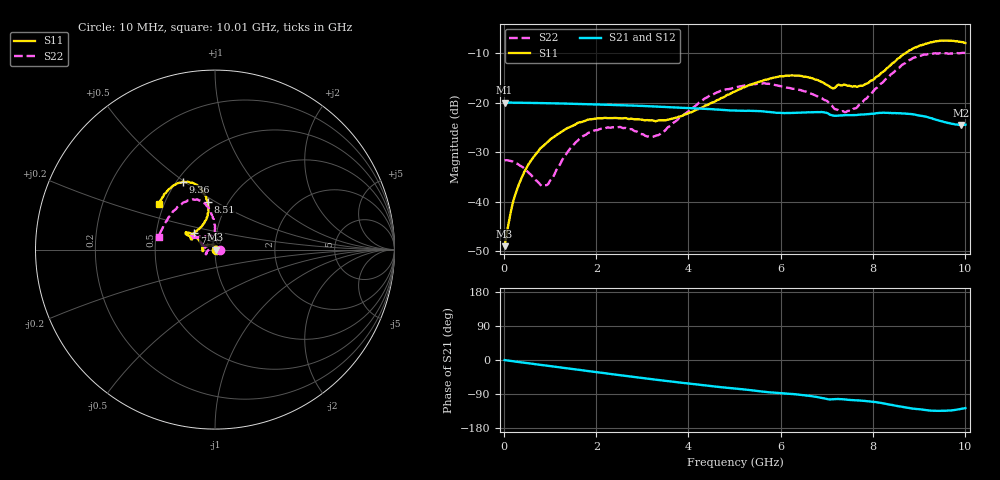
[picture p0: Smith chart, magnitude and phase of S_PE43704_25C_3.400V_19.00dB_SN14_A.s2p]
! Device ID: PE43704
! Dir: z:\PE43704\PE43704_Char_1_20130516\PE43704\AMB\3p400V\19p00dB
! Serial: 14
! Insertion: A
! Impedance: 50 ohm
! Temp: Amb
! VDD: 3.400V
! Attenuation Step: 19.00dB
! IDD: 1.140463e-01mA
#  Hz  S  RI  R  50
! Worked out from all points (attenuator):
!   401 points, 10 MHz to 10.01 GHz, reference 50 ohm
!   highest |S21| = -19.96 dB at 10 MHz (marker M1); lowest = -24.5 dB at 9.91 GHz (marker M2)
!   lowest |S11| = -49.0 dB at 10 MHz (marker M3), VSWR 1.01, Z = 50.4 + j0.047 ohm
!   |S11| at or under -10 dB: start of sweep to 8.714 GHz
!   |S22| runs from -36.9 to -9.9 dB; largest |S21 - S12| = 0.0012
!   S11 on the Smith chart (normalised r, x): 10 MHz: 1.01, +0.00; 7.46 GHz: 0.78, +0.15; 8.51 GHz: 0.81, +0.46; 9.36 GHz: 0.54, +0.49; 10.01 GHz: 0.47, +0.28
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1e7  0.00352 0.000467  0.1005 -0.000334  0.1005 -0.000251  0.0261 0.000237
2.35e8  0.00173 0.0114  0.0999 -0.00701  0.0999 -0.00697  0.0237 0.0071
5.6e8  -0.00776 0.0238  0.0983 -0.0161  0.0982 -0.0161  0.0133 0.0138
8.1e8  -0.0198 0.0293  0.0964 -0.0229  0.0964 -0.0229  0.000923 0.0145
9.35e8  -0.0261 0.0297  0.0953 -0.0262  0.0953 -0.0261  -0.00619 0.0134
1.385e9  -0.0504 0.024  0.0903 -0.0375  0.0904 -0.0375  -0.0321 0.00166
1.685e9  -0.062 0.0152  0.0862 -0.0445  0.0863 -0.0445  -0.0441 -0.00997
2.385e9  -0.0699 -0.00424  0.0747 -0.0585  0.0747 -0.0585  -0.0507 -0.0253
3.36e9  -0.0664 -0.000702  0.0549 -0.0728  0.055 -0.0727  -0.0473 0.00192
4.385e9  -0.084 0.0429  0.0334 -0.0801  0.0334 -0.0802  -0.0947 0.0598
5.01e9  -0.1083 0.0719  0.0212 -0.0807  0.0213 -0.0806  -0.1224 0.0733
5.96e9  -0.1565 0.0955  0.00392 -0.079  0.0042 -0.0789  -0.128 0.0741
6.685e9  -0.1565 0.0818  -0.00812 -0.0797  -0.00818 -0.0797  -0.1011 0.0688
7.11e9  -0.1258 0.0647  -0.0178 -0.0726  -0.0179 -0.0726  -0.0565 0.0747
7.46e9  -0.1148 0.094  -0.0194 -0.0724  -0.0191 -0.0725  -0.0217 0.0798
7.835e9  -0.0684 0.1379  -0.024 -0.0726  -0.024 -0.0725  -0.0016 0.1084
8.36e9  -0.0366 0.2304  -0.0363 -0.0697  -0.0363 -0.0704  -0.0129 0.185
8.51e9  -0.0394 0.2657  -0.0401 -0.0672  -0.04 -0.0677  -0.025 0.2137
8.935e9  -0.0897 0.3513  -0.0479 -0.0584  -0.0474 -0.0581  -0.0897 0.2745
9.36e9  -0.1789 0.3778  -0.047 -0.0484  -0.0471 -0.0484  -0.1807 0.2598
9.91e9  -0.2951 0.2859  -0.0376 -0.0462  -0.0379 -0.046  -0.297 0.1105
1.001e10  -0.312 0.2527  -0.0361 -0.0478  -0.0368 -0.0481  -0.3118 0.0694
